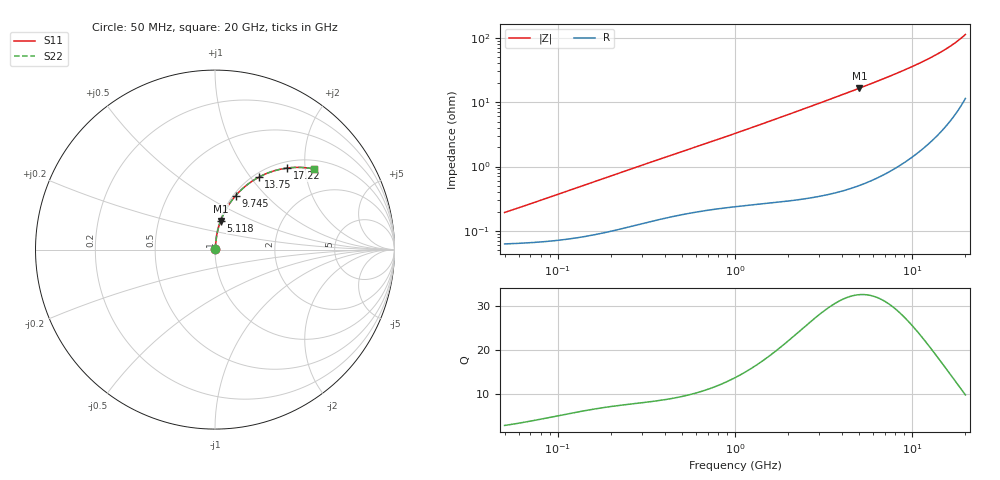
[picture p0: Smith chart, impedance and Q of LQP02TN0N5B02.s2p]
!Murata Part Number: LQP02TN0N5B02
!These Parameters are Measured in Series Mode Connection
!  o--[Z]--o
!Port1  Port2
!  o-------o
!Freq. Start=50[MHz] Stop=20[GHz], 401[Steps]
# Hz S RI R 50
!Freq.(Hz) S11(Real) S11(Imag) S21(Real) S21(Imag) S12(Real) S12(Imag) S22(Real) S22(Imag)
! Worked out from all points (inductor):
!   401 points, 50 MHz to 20 GHz, reference 50 ohm
!   read as one part in series: L = 581 pH near 52.3 MHz
!   highest Q = 32.5 at 5.041 GHz (marker M1), where L = 520 pH
!   S11 on the Smith chart (normalised r, x): 50 MHz: 1.00, +0.00; 5.118 GHz: 1.01, +0.33; 9.745 GHz: 1.03, +0.69; 13.75 GHz: 1.06, +1.10; 17.22 GHz: 1.12, +1.61; 20 GHz: 1.23, +2.24
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5e7  0.00063 0.00183  0.9994 -0.00183  0.9994 -0.00183  0.00063 0.00183
6.646115e7  0.000656 0.00242  0.9993 -0.00242  0.9993 -0.00242  0.000656 0.00242
1.364002e8  0.000826 0.00492  0.9992 -0.00492  0.9992 -0.00492  0.000826 0.00492
3.721004e8  0.00166 0.0127  0.9983 -0.0127  0.9983 -0.0127  0.00166 0.0127
1e9  0.00342 0.0323  0.9966 -0.0323  0.9966 -0.0323  0.00342 0.0323
1.714689e9  0.00577 0.0546  0.9942 -0.0546  0.9942 -0.0546  0.00577 0.0546
2.728004e9  0.0108 0.0864  0.9892 -0.0864  0.9892 -0.0864  0.0108 0.0864
3.736399e9  0.0181 0.118  0.9819 -0.118  0.9819 -0.118  0.0181 0.118
5.041459e9  0.0311 0.1588  0.9689 -0.1588  0.9689 -0.1588  0.0311 0.1588
5.117541e9  0.032 0.1612  0.968 -0.1612  0.968 -0.1612  0.032 0.1612
6.217679e9  0.0464 0.1953  0.9536 -0.1953  0.9536 -0.1953  0.0464 0.1953
7.442007e9  0.0663 0.2328  0.9337 -0.2328  0.9337 -0.2328  0.0663 0.2328
8.516016e9  0.0872 0.2651  0.9128 -0.2651  0.9128 -0.2651  0.0872 0.2651
9.745021e9  0.1156 0.3011  0.8844 -0.3011  0.8844 -0.3011  0.1156 0.3011
1.166392e10  0.1698 0.3538  0.8302 -0.3538  0.8302 -0.3538  0.1698 0.3538
1.276073e10  0.2067 0.3811  0.7933 -0.3811  0.7933 -0.3811  0.2067 0.3811
1.375312e10  0.2439 0.4035  0.7561 -0.4035  0.7561 -0.4035  0.2439 0.4035
1.550395e10  0.3186 0.4354  0.6814 -0.4354  0.6814 -0.4354  0.3186 0.4354
1.721783e10  0.402 0.4543  0.598 -0.4543  0.598 -0.4543  0.402 0.4543
1.828096e10  0.4581 0.4582  0.5419 -0.4582  0.5419 -0.4582  0.4581 0.4582
1.940974e10  0.5203 0.4544  0.4797 -0.4544  0.4797 -0.4544  0.5203 0.4544
2e10  0.5535 0.4488  0.4465 -0.4488  0.4465 -0.4488  0.5535 0.4488
